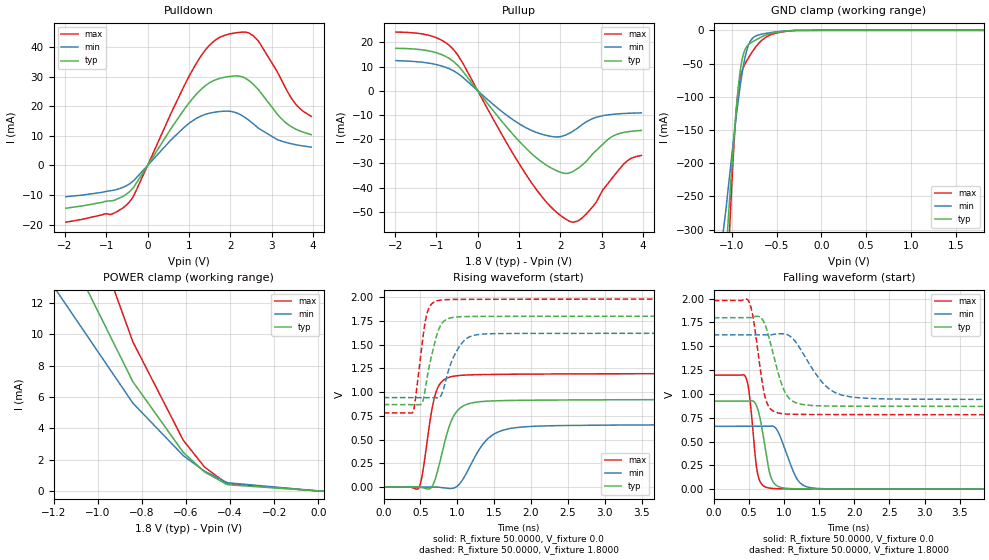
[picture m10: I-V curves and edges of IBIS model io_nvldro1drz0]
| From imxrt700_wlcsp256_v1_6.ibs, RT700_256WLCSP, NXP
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[Model] io_nvldro1drz0
|   Model io_nvldro1drz0
| This model was characterised for following simulation conditions:
| External (pad) voltage:
|   - Typ: 1.8V,   - Min: 1.62V,   - Max: 1.98V
| Library cells for typ/min/max conditions are connected as defined below:
|  ipp_io - External Pad
|  ipp_do - Core Input
|  ipp_obe - Output Buffer Enable
|  config1v21v8 - gnde
|  drive0 - gnd
|  drive1 - vdd
|  gnd - gnd
|  gnde - gnde
|  ncgather - NC
|  vdd - vdd
|  vdde1v8 - vdde1v8
| All other pins connected to ground
Model_type I/O
Polarity   Non-Inverting
Enable   Active-Low
Vinl =   0.5400V
Vinh =   1.2600V
Vmeas =  0.9000V
Cref =   30.0000pF
Rref =   1.0000M
Vref =   1.8000V
C_comp   2.6153pF   2.5662pF   2.7105pF
|C_comp_pullup   1.3378pF   1.3962pF   1.2821pF
|C_comp_pulldown   0.0F   0.0F   0.0F
[Model Spec]
| variable   typ   min   max
Vinh   1.2600V   NA   NA
Vinl   0.5400V   NA   NA
Vref   1.8000V   1.8000V   1.8000V
Cref   30.0000pF   30.0000pF   30.0000pF
Rref   1.0000M   1.0000M   1.0000M
[Temperature Range]   25.0000   0.1250k   -40.0000
[Voltage Range]   1.8000V   1.6200V   1.9800V
[Pullup Reference]   1.8000V   1.6200V   1.9800V
[Pulldown Reference]   0.0V   0.0V   0.0V
[POWER Clamp Reference]   1.8000V   1.6200V   1.9800V
[GND Clamp Reference]   0.0V   0.0V   0.0V
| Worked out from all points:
|   slope of the pulldown table from 0 to 0.27 V, typ, clamps not added: 45.3 ohm
|   slope of the pullup table from 0 to 0.27 V, typ, clamps not added: 45.3 ohm
|   GND clamp passes 1 mA (typ) near -0.39 V on its own axis
|   POWER clamp passes 1 mA (typ) near -0.49 V on its own axis
|   rising waveform, R_fixture 50.0000, V_fixture 0.0: 20-80 % time 207ps typ, 329ps min, 148ps max; typ from 0 V to 0.924 V
|   rising waveform, R_fixture 50.0000, V_fixture 1.8000: 20-80 % time 157ps typ, 203ps min, 118ps max; typ from 0.868 V to 1.8 V
|   falling waveform, R_fixture 50.0000, V_fixture 0.0: 20-80 % time 130ps typ, 207ps min, 93.6ps max; typ from 0.924 V to 0 V
|   falling waveform, R_fixture 50.0000, V_fixture 1.8000: 20-80 % time 212ps typ, 381ps min, 140ps max; typ from 1.8 V to 0.868 V
[Pulldown]
|Voltage   I(typ)   I(min)   I(max)
-1.98V    -14.44mA   -10.56mA   -19.16mA
-876mV    -11.95mA   -8.474mA   -16.47mA
-432mV    -8.785mA   -6.156mA   -12.17mA
1.056V    22.06mA    14.79mA    31.49mA
1.428V    27.27mA    17.41mA    39.54mA
1.788V    29.59mA    18.28mA    43.57mA
2.232V    30.17mA    17.27mA    44.99mA
2.568V    27.29mA    13.96mA    43.71mA
2.688V    25.52mA    12.55mA    41.94mA
3.288V    15.12mA    8.036mA    27.57mA
3.6V      12.2mA     6.986mA    20.49mA
3.96V     10.43mA    6.219mA    16.61mA
[Pullup]
|Voltage   I(typ)   I(min)   I(max)
-1.98V    17.57mA    12.48mA    24.28mA
-1.104V   16.21mA    11.21mA    22.58mA
-588mV    12.13mA    8.275mA    17.1mA
576mV     -12.48mA   -8.454mA   -17.83mA
1.14V     -23.29mA   -15.01mA   -33.86mA
1.704V    -31.18mA   -18.6mA    -46.8mA
2.22V     -33.94mA   -17.52mA   -53.9mA
2.412V    -32.21mA   -15.49mA   -53.9mA
2.628V    -29.18mA   -12.8mA    -50.92mA
3.228V    -19.16mA   -9.795mA   -36.63mA
3.66V     -16.86mA   -9.286mA   -28.45mA
3.96V     -16.39mA   -9.132mA   -26.7mA
[GND_clamp]
|Voltage   I(typ)   I(min)   I(max)
-1.98V    -2.304A    -1.314A    -3.648A
-1.188V   -579.3mA   -402.9mA   -809.8mA
-1.068V   -345.9mA   -273.9mA   -436.6mA
-1.02V    -246.9mA   -214.1mA   -290.1mA
-972mV    -156.3mA   -155.7mA   -166mA
-924mV    -82.86mA   -102.6mA   -86.85mA
-864mV    -33.43mA   -49.36mA   -54.12mA
-816mV    -21.98mA   -23.37mA   -42.16mA
-744mV    -15.43mA   -9.445mA   -27.16mA
-588mV    -5.426mA   -3.899mA   -8.058mA
-312mV    -266.2uA   -304.2uA   -358.5uA
1.812V    32.97nA    19.96uA    18.44nA
[POWER_clamp]
|Voltage   I(typ)   I(min)   I(max)
-1.98V    42.79mA    32.01mA    58.17mA
-1.356V   21.6mA     16.3mA     29.63mA
-840mV    6.97mA     5.605mA    9.513mA
-612mV    2.467mA    2.258mA    3.244mA
-516mV    1.219mA    1.266mA    1.533mA
-420mV    455.4uA    582uA      529uA
-408mV    393.4uA    518.7uA    452.7uA
0V        28.12nA    179.8nA    22.83nA
24mV      22.85nA    114.4nA    21.08nA
[Ramp]
| variable   typ   min   max
dV/dt_r  0.5543/0.2068n   0.3958/0.3283n   0.7181/0.1477n
dV/dt_f  0.5589/0.2122n   0.4069/0.3804n   0.7194/0.1398n
R_load = 50.0000
[Rising Waveform]
R_fixture= 50.0000
V_fixture= 0.0
V_fixture_min= 0.0
V_fixture_max= 0.0
|time   V(typ)   V(min)   V(max)
0s        245.2nV    2.644uV    458.4nV
476.8ps   -388.8uV   2.89uV     -10.7mV
527.6ps   -7.912mV   3.92uV     143mV
642ps     -9.138mV   -4.406uV   760.3mV
749.3ps   219.3mV    -2.683mV   1.068V
941ps     733.4mV    -13.21mV   1.166V
1.245ns   892.6mV    326.1mV    1.183V
1.666ns   910.9mV    607.8mV    1.188V
2.943ns   918.5mV    651.3mV    1.193V
60ns      923.8mV    659.6mV    1.197V
[Rising Waveform]
R_fixture= 50.0000
V_fixture= 1.8000
V_fixture_min= 1.6200
V_fixture_max= 1.9800
|time   V(typ)   V(min)   V(max)
0s        868.4mV    941.8mV    780.9mV
396.8ps   868.5mV    941.8mV    789.9mV
426.3ps   868.4mV    941.8mV    894.7mV
521.7ps   885.3mV    941.8mV    1.505V
595.3ps   1.175V     941.8mV    1.846V
744.4ps   1.654V     941.2mV    1.965V
889.2ps   1.777V     1.252V     1.975V
1.132ns   1.796V     1.568V     1.977V
1.643ns   1.798V     1.617V     1.978V
60ns      1.8V       1.62V      1.98V
[Falling Waveform]
R_fixture= 50.0000
V_fixture= 0.0
V_fixture_min= 0.0
V_fixture_max= 0.0
|time   V(typ)   V(min)   V(max)
0s        923.8mV    659.6mV    1.197V
452.2ps   923.7mV    659.6mV    1.179V
506.5ps   923.3mV    659.6mV    996.7mV
598.3ps   891.7mV    659.6mV    288.2mV
638.2ps   807.6mV    659.6mV    119.3mV
795.2ps   168.8mV    660mV      10.94mV
922.5ps   26.29mV    591mV      4.569mV
1.215ns   3.522mV    76.44mV    2.817mV
1.647ns   2.131mV    3.574mV    2.262mV
60ns      581.2nV    6.585uV    485.4nV
[Falling Waveform]
R_fixture= 50.0000
V_fixture= 1.8000
V_fixture_min= 1.6200
V_fixture_max= 1.9800
|time   V(typ)   V(min)   V(max)
0s        1.8V       1.62V      1.98V
493.9ps   1.8V       1.62V      1.977V
562.6ps   1.809V     1.62V      1.792V
679.1ps   1.794V     1.62V      1.171V
801.7ps   1.547V     1.62V      847.4mV
977.8ps   1.078V     1.632V     792.6mV
1.125ns   922.9mV    1.581V     786.3mV
1.693ns   872.3mV    1.028V     783.2mV
2.558ns   870mV      946.3mV    782.4mV
60ns      868.4mV    941.8mV    780.9mV
